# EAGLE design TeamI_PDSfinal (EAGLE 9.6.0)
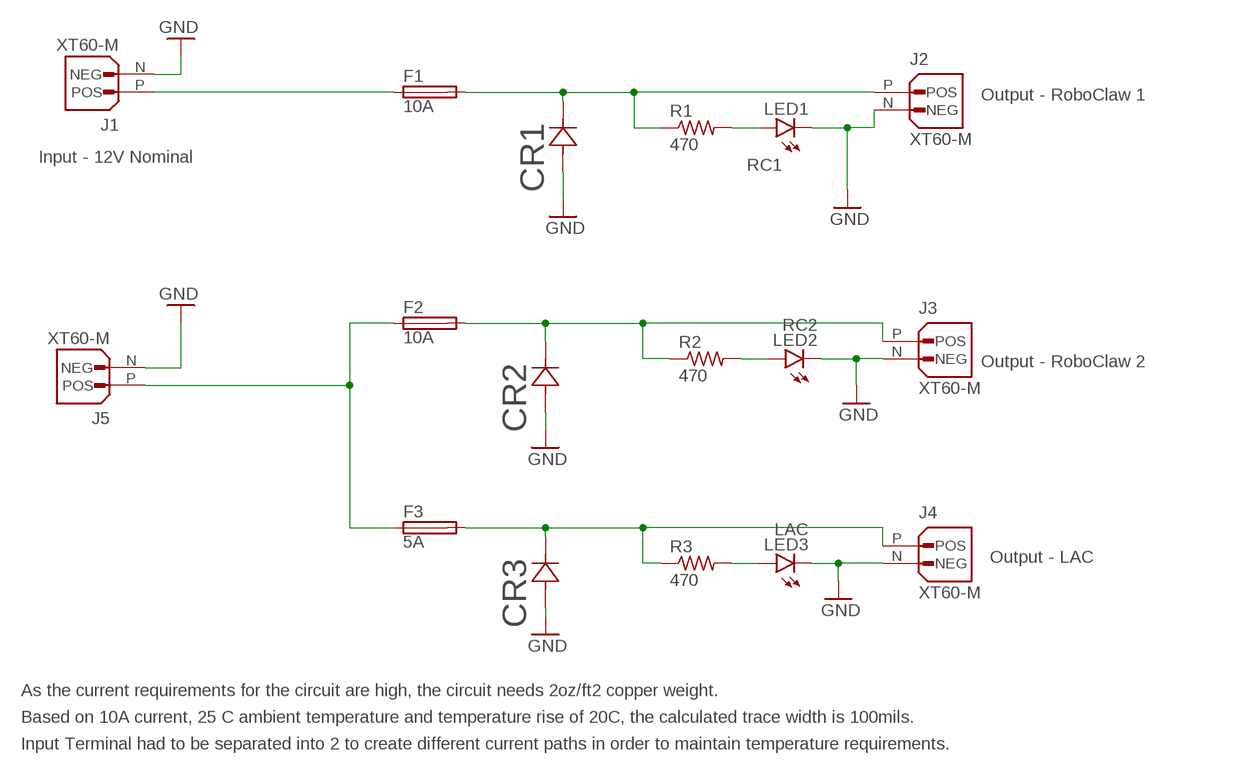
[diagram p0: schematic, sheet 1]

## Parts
CR1  P4SMA16A  [P4SMASERIES_LTF]
CR2  P4SMA16A  [P4SMASERIES_LTF]
CR3  P4SMA16A  [P4SMASERIES_LTF]
F1  10A  TR5  [TR5]
F2  10A  TR5  [TR5]
F3  5A  TE5  [TE5]
J1  XT60-M  [AMASS_XT60-M]
J2  XT60-M  [AMASS_XT60-M]
J3  XT60-M  [AMASS_XT60-M]
J4  XT60-M  [AMASS_XT60-M]
J5  XT60-M  [AMASS_XT60-M]
LED1  RC1  LEDSMT1206  [1206]
LED2  RC2  LEDSMT1206  [1206]
LED3  LAC  LEDSMT1206  [1206]
R1  470  R-US_R1206  [R1206]
R2  470  R-US_R1206  [R1206]
R3  470  R-US_R1206  [R1206]

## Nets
GND: CR1.2 CR2.2 CR3.2 J1.N(NEG) J2.N(NEG) J3.N(NEG) J4.N(NEG) J5.N(NEG) LED1.C LED2.C LED3.C
N$1: CR1.1 F1.2 J2.P(POS) R1.1
N$3: CR3.1 F3.2 J4.P(POS) R3.1
N$4: LED1.A R1.2
N$5: F1.1 J1.P(POS)
N$6: CR2.1 F2.2 J3.P(POS) R2.1
N$7: LED2.A R2.2
N$9: LED3.A R3.2
N$14: F2.1 F3.1 J5.P(POS)

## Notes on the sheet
- Output - RoboClaw 1
- Input - 12V Nominal
- Output - RoboClaw 2
- Output - LAC
- As the current requirements for the circuit are high, the circuit needs 2oz/ft2 copper weight.
- Based on 10A current, 25 C ambient temperature and temperature rise of 20C, the calculated trace width is 100mils.
- Input Terminal had to be separated into 2 to create different current paths in order to maintain temperature requirements.

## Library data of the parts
CR1-CR3 = P4SMA16A:P4SMA16A; COPYRIGHT: Copyright (C) 2025 Ultra Librarian. All rights reserved.; MANUFACTURER_PART_NUMBER: P4SMA16A; MFR_NAME: Littelfuse Inc
F1 F2 = fuse:TR5: FUSE; OC_FARNELL: unknown; OC_NEWARK: unknown
F3 = fuse:TE5: FUSE; OC_FARNELL: unknown; OC_NEWARK: unknown
J1-J5 = XT60-M:XT60-M: Check availability; AVAILABILITY: Not in stock; CHECK_PRICES: https://www.snapeda.com/parts/XT60-M/AMASS/view-part/?ref=eda; DESCRIPTION: Plug; DC supply; XT60; male; PIN: 2; for cable; soldered; 30A; 500V; MF: AMASS; MP: XT60-M; PACKAGE: Package; PRICE: None; SNAPEDA_LINK: https://www.snapeda.com/parts/XT60-M/AMASS/view-part/?ref=snap
LED1-LED3 = led:LED: LED
R1-R3 = rcl:R-US_: RESISTOR, American symbol; SPICEPREFIX: R

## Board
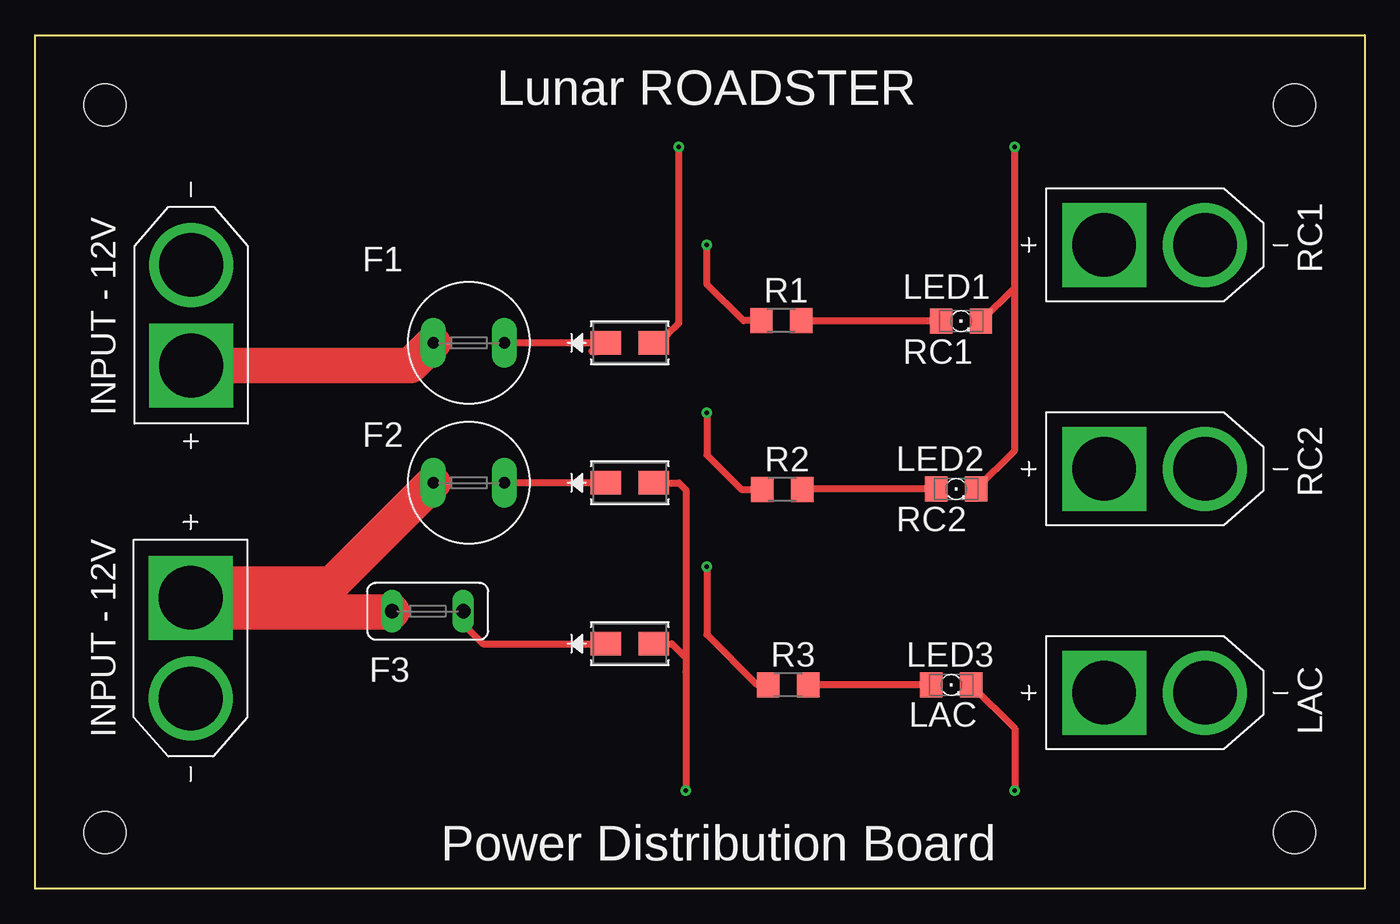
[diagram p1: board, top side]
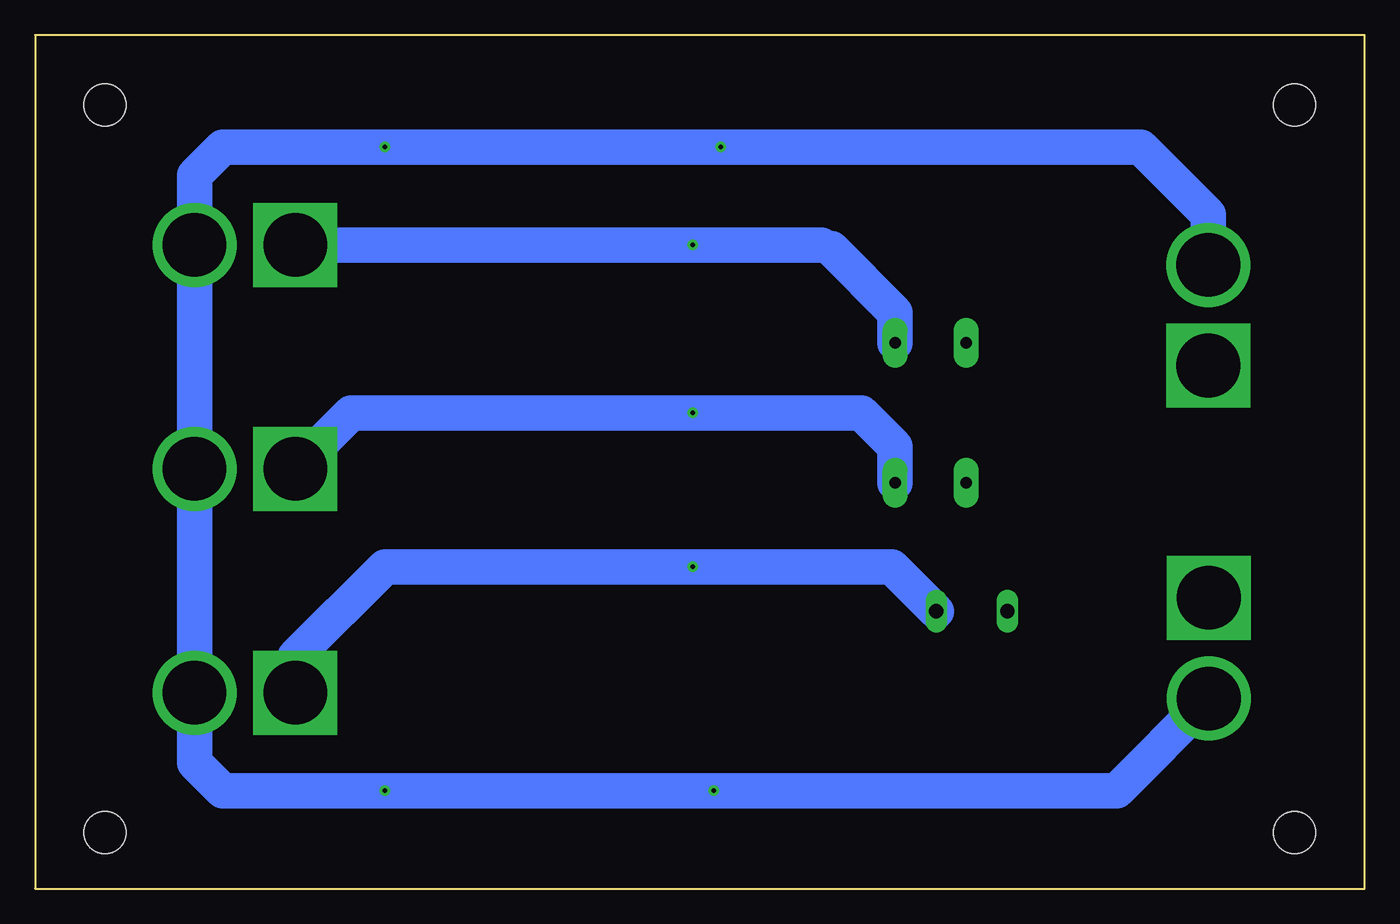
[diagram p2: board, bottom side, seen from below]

Size 95 x 61 mm. Coordinates in mm from the lower left corner, seen from the top.
Outline: 0,61 95,61 95,0 0,0 0,61
Copper layers (1*16): Top 0.035mm / dielectric 1.5mm / Bottom 0.035mm
Design rules "default *": minimum track width 20mil, minimum drill 0.35mm, track to track 6mil, track to pad 6mil, pad to pad 6mil, via to via 6mil, smd to smd 6mil, copper to edge 40mil, drill to drill 6mil, minimum pad ring 10mil, minimum via ring 8mil, stop-mask expansion 4mil, vias tented up to drill 0mil, thermal gap 10mil
Holes 3 mm at 5,56 5,4 90,4 90,56

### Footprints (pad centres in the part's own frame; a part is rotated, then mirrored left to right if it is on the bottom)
P4SMASERIES_LTF = smd 2.184 x 1.651: 1 -1.702,0; 2 1.702,0
TR5 = drill 0.813 pad 1.778 long: 1 -2.54,0; 2 2.54,0
TE5 = drill 1.016 long: 1 -2.54,0; 2 2.54,0
AMASS_XT60-M = drill 4.55 pad 6: N 3.6,0 | drill 4.55 pad 6 square: P -3.6,0
1206 = smd 1.6 x 1.803: A -1.422,0; C 1.422,0
R1206 = smd 1.6 x 1.803: 1 -1.422,0; 2 1.422,0

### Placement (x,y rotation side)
CR1  42.5,39 0 top
CR2  42.5,29 0 top
CR3  42.5,17.5 0 top
F1  31,39 0 top
F2  31,29 0 top
F3  28.06,19.82 0 top
J1  11.16,40.97 90 top
J2  80,46 0 top
J3  80,30 0 top
J4  80,14 0 top
J5  11.12,17.18 270 top
LED1  66.17,40.55 0 top
LED2  65.82,28.55 0 top
LED3  65.47,14.55 0 top
R1  53.33,40.59 0 top
R2  53.39,28.52 0 top
R3  53.82,14.56 0 top

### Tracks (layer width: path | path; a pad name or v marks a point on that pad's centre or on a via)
GND  (via drill 0.35)
  Top 0.508: LED1.C 70,42.96 | 70,42.96 v70,53 | LED2.C 70,31.31 70,42.96 | LED3.C 70,11.44 v70,7 | CR1.2 44.81,39.61 45.2,39.61 46,40.41 v46,53 | CR3.2 45.5,17.5 46.5,16.5 | 46.5,16.5 46.5,15.5 v46.5,7 | CR2.2 46,29 46.5,28.5 46.5,16.5
  Bottom 2.54: J1.N 11.16,48.16 16,53 v46,53 v70,53 81.6,53 83.6,51 J2.N J3.N J4.N 83.6,9 81.6,7 v70,7 v46.5,7 17.7,7 J5.N
N$1  (via drill 0.35)
  Top 0.508: R1.1 50.63,40.59 48,43.21 v48,46 | v48,46 | 39.8,38.39 40.19,38.39 CR1.1 F1.2
  Bottom 0.508: 38.81,46 38.38,46 38.1,45.72
  Bottom 2.54: 38.81,46 v48,46 J2.P | F1.2 33.54,41.16 38.1,45.72
N$3  (via drill 0.35)
  Top 0.508: v48,23 48,18.16 51.6,14.56 R3.1 | F3.2 30.6,18.9 32,17.5 CR3.1
  Bottom 2.54: F3.2 33.78,23 v48,23 70,23 76.4,16.6 J4.P
N$4
  Top 0.508: R1.2 54.79,40.55 LED1.A
N$5
  Top 2.54: F1.1 26.83,37.37 J1.P
N$6  (via drill 0.35)
  Top 0.508: v48,34 48,31 50.48,28.52 R2.1 | 40.62,28.82 CR2.1 F2.2
  Bottom 2.54: J3.P 72.4,34 v48,34 35.94,34 33.54,31.6 F2.2
N$7
  Top 0.508: LED2.A 54.84,28.55 R2.2
N$9
  Top 0.508: R3.2 LED3.A
N$14
  Top 0.508: 24.48,25.02
  Top 2.54: F3.1 25.48,19.78 12.12,19.78 J5.P 12.12,21.78 16.64,21.78 21.24,21.78 24.48,25.02 F2.1

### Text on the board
tNames: Lunar ROADSTER | INPUT - 12V | RC1 | RC1 | RC2 | RC2 | INPUT - 12V | LAC | LAC | Power Distribution Board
